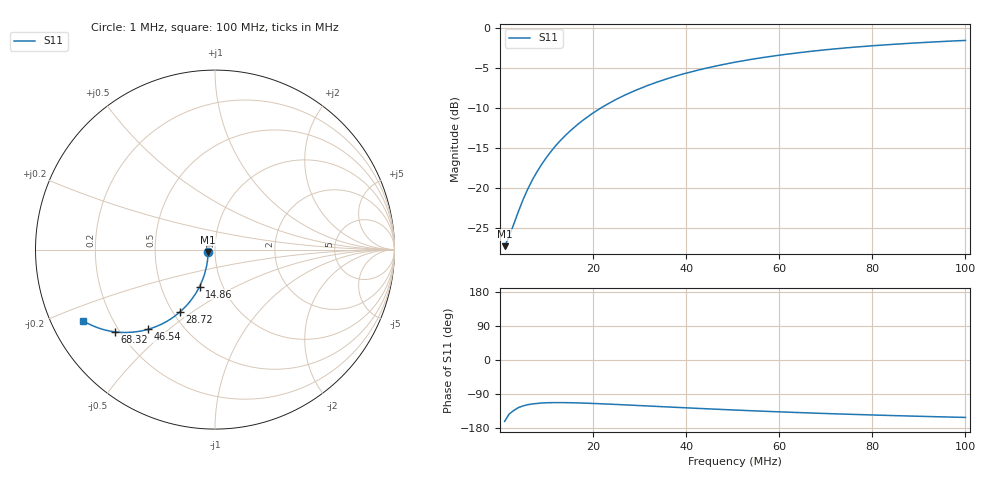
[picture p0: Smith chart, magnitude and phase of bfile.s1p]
# Hz S RI R 50.0
! written by SimSmith version 18.3b
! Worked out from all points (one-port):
!   101 points, 1 MHz to 100 MHz, reference 50 ohm
!   lowest |S11| = -27.3 dB at 1 MHz (marker M1), VSWR 1.09, Z = 46.1 - j1.23 ohm
!   |S11| at or under -10 dB: start of sweep to 21.77 MHz
!   S11 on the Smith chart (normalised r, x): 1 MHz: 0.92, -0.02; 14.86 MHz: 0.78, -0.34; 28.72 MHz: 0.54, -0.45; 46.54 MHz: 0.32, -0.43; 68.32 MHz: 0.18, -0.35; 100 MHz: 0.10, -0.25
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1000000  -0.0409 -0.0133
1990000  -0.0393 -0.0302
3970000  -0.0412 -0.0578
4960000  -0.0436 -0.0719
5950000  -0.0458 -0.0862
6940000  -0.0488 -0.1002
7930000  -0.0524 -0.1139
9910000  -0.0597 -0.1412
1.189e7  -0.0694 -0.168
1.387e7  -0.0801 -0.1937
1.486e7  -0.0863 -0.2059
1.684e7  -0.099 -0.2302
1.981e7  -0.121 -0.2642
2.278e7  -0.1447 -0.2955
2.575e7  -0.1705 -0.3239
2.872e7  -0.1976 -0.3493
3.367e7  -0.2449 -0.3856
3.862e7  -0.2938 -0.4137
4.258e7  -0.3327 -0.4305
4.654e7  -0.3705 -0.4434
5.05e7  -0.4082 -0.4526
5.644e7  -0.461 -0.4603
6.337e7  -0.5182 -0.4609
6.832e7  -0.5564 -0.4581
7.525e7  -0.6038 -0.4501
8.119e7  -0.6401 -0.4399
8.812e7  -0.678 -0.4254
1e8  -0.7328 -0.3977
